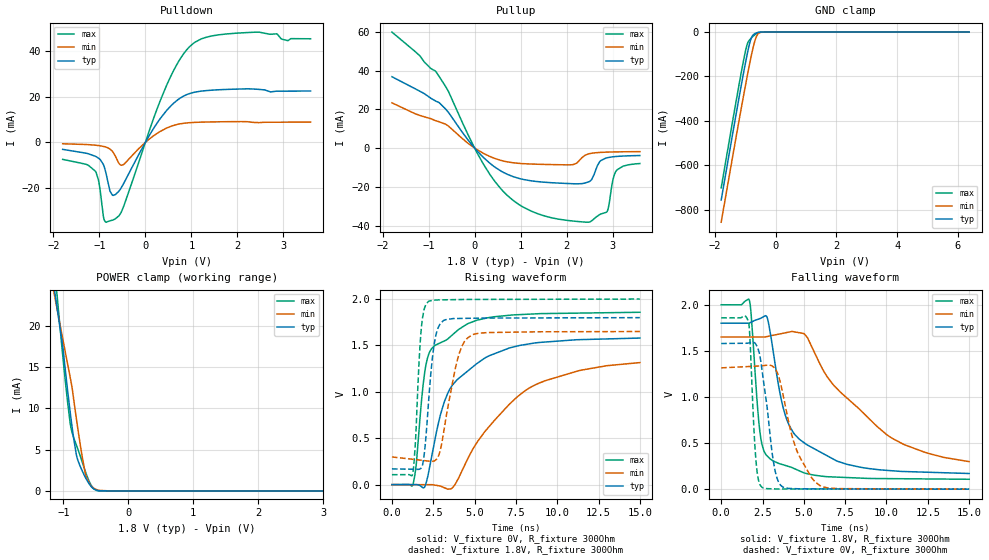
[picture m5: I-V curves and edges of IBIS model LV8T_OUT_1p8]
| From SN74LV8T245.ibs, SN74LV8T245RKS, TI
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[Model]   LV8T_OUT_1p8
Model_type   I/O
Polarity   Non-Inverting
Enable   Active-Low
Vinl = 0.51
Vinh = 1.1
Vmeas = 0.9
Vref = 0
Cref = 2pF
Rref = 100000
|   typ   min   max
C_comp   6.7pF   6.5pF   7pF
[Voltage Range]   1.8   1.65   2
[Temperature Range]   25   125   -40
[Pullup Reference]   1.8   1.65   2
[Pulldown Reference]   0   0   0
[Power Clamp Reference]   1.8   1.65   2
[GND Clamp Reference]   0   0   0
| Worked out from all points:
|   slope of the pulldown table from 0 to 0.27 V, typ, clamps not added: 30.3 ohm
|   slope of the pullup table from 0 to 0.27 V, typ, clamps not added: 41.2 ohm
|   GND clamp passes 1 mA (typ) near -0.56 V on its own axis
|   POWER clamp passes 1 mA (typ) near -0.61 V on its own axis
|   falling waveform, V_fixture 1.8V, R_fixture 300Ohm: 20-80 % time 1.91ns typ, 4.28ns min, 546ps max; typ from 1.8 V to 0.17 V
|   rising waveform, V_fixture 0V, R_fixture 300Ohm: 20-80 % time 2.44ns typ, 3.87ns min, 971ps max; typ from 0 V to 1.58 V
|   rising waveform, V_fixture 1.8V, R_fixture 300Ohm: 20-80 % time 477ps typ, 882ps min, 317ps max; typ from 0.17 V to 1.8 V
|   falling waveform, V_fixture 0V, R_fixture 300Ohm: 20-80 % time 656ps typ, 1.31ns min, 299ps max; typ from 1.58 V to 0 V
[Pulldown]
|   Voltage   I(typ)   I(min)   I(max)
-1.796V   -3.045mA   -600uA     -7.42mA
-1.083V   -6.104mA   -1.23mA    -12.66mA
-1.009V   -7.035mA   -1.406mA   -17.51mA
-893.5mV  -10.69mA   -1.841mA   -33.97mA
-767.5mV  -21.4mA    -2.913mA   -34.28mA
-694mV    -23.17mA   -4.51mA    -33.86mA
-473.5mV  -18.04mA   -9.675mA   -28.07mA
324.5mV   10.45mA    4.819mA    18.3mA
618.5mV   17.21mA    7.455mA    31.63mA
954.5mV   21.33mA    8.616mA    41.74mA
1.962V    23.3mA     9.091mA    47.75mA
3.59V     22.5mA     8.877mA    45.34mA
[GND Clamp]
|   Voltage   I(typ)   I(min)   I(max)
-1.796V   -756.6mA   -856.2mA   -701.6mA
-1.188V   -279.6mA   -382.9mA   -221.3mA
-1.072V   -193.2mA   -296.1mA   -136.2mA
-988mV    -132.9mA   -234.2mA   -80.47mA
-914.5mV  -83.48mA   -181.5mA   -46.74mA
-851.5mV  -47.24mA   -137.9mA   -33.82mA
-799mV    -25.51mA   -103.2mA   -26.25mA
-683.5mV  -6.635mA   -38.29mA   -11.53mA
-631mV    -3.444mA   -18.64mA   -6.502mA
-568mV    -1.185mA   -5.967mA   -2.299mA
-274mV    -10.31nA   -2.458uA   0A
6.372V    0A         0A         0A
[Pullup]
|   Voltage   I(typ)   I(min)   I(max)
-1.796V   36.82mA    23.35mA    59.86mA
-841mV    24.17mA    14.08mA    39.43mA
324.5mV   -7.713mA   -4.277mA   -13.36mA
702.5mV   -13.49mA   -7.102mA   -24.3mA
1.081V    -16.33mA   -8.097mA   -30.81mA
2.131V    -18.42mA   -8.573mA   -37.67mA
2.509V    -17.08mA   -2.833mA   -38.09mA
2.719V    -7.037mA   -2.275mA   -34.36mA
2.886V    -4.992mA   -2.098mA   -32.39mA
3.002V    -4.533mA   -2.025mA   -16.75mA
3.075V    -4.357mA   -1.99mA    -11.82mA
3.59V     -3.877mA   -1.859mA   -7.992mA
[POWER Clamp]
|   Voltage   I(typ)   I(min)   I(max)
-1.796V   61.45mA    51.6mA     74.22mA
-1.188V   27.14mA    25.88mA    30.08mA
-1.103V   22.6mA     22.36mA    24.31mA
-1.093V   22.04mA    21.92mA    23.5mA
-1.009V   17.53mA    18.45mA    16.44mA
-967mV    14.55mA    16.74mA    13.18mA
-883mV    8.87mA     13.32mA    7.694mA
-799mV    4.394mA    8.8mA      5.562mA
-662.5mV  1.684mA    2.226mA    2.411mA
-599.5mV  831uA      918.6uA    1.136mA
-484mV    74.52uA    145.8uA    53.97uA
6.372V    0A         0A         0A
[Ramp]
R_load = 300
|   typ   min   max
dV/dt_r   0.947756/2.43296e-09   0.789158/3.87689e-09   1.11451/9.59874e-10
dV/dt_f   0.977899/1.90392e-09   0.810908/4.28098e-09   1.13551/5.4593e-10
[Falling Waveform]
V_fixture = 1.8V
V_fixture_min = 1.65V
V_fixture_max = 2V
R_fixture = 300Ohm
C_fixture = 0F
|   Time   V(typ)   V(min)   V(max)
0s        1.8V       1.65V      2V
1.701ns   1.801V     1.65V      2.051V
2.357ns   1.851V     1.65V      603mV
2.733ns   1.878V     1.654V     369.1mV
2.975ns   1.689V     1.663V     326.5mV
3.926ns   776.4mV    1.697V     254.8mV
5.125ns   489.2mV    1.664V     171.1mV
6.735ns   330.7mV    1.142V     132.8mV
9.983ns   204.4mV    595.9mV    114.5mV
15ns      169.8mV    298.5mV    107.3mV
[Rising Waveform]
V_fixture = 0V
V_fixture_min = 0V
V_fixture_max = 0V
R_fixture = 300Ohm
C_fixture = 0F
|   Time   V(typ)   V(min)   V(max)
0s        101.7uV    1.708uV    32.48uV
1.269ns   589.5uV    -297.5uV   -85.04uV
1.466ns   665.3uV    -344uV     208.2mV
1.993ns   -20.9mV    -468.3uV   1.222V
2.568ns   452.4mV    -4.419mV   1.495V
2.95ns    762.7mV    -16.71mV   1.53V
3.531ns   1.038V     -46.61mV   1.594V
5.855ns   1.387V     620.6mV    1.8V
8.786ns   1.53V      1.085V     1.841V
15ns      1.58V      1.315V     1.858V
[Rising Waveform]
V_fixture = 1.8V
V_fixture_min = 1.65V
V_fixture_max = 2V
R_fixture = 300Ohm
C_fixture = 0F
|   Time   V(typ)   V(min)   V(max)
0s        169.8mV    298.5mV    107.3mV
1.257ns   165.8mV    273.2mV    116.4mV
1.423ns   165.3mV    269.8mV    460.7mV
1.77ns    180.2mV    262.8mV    1.668V
2.195ns   840.2mV    254.3mV    1.972V
2.487ns   1.422V     252.5mV    1.986V
2.787ns   1.688V     297.9mV    1.991V
4ns       1.791V     1.371V     1.994V
4.809ns   1.793V     1.61V      1.996V
15ns      1.8V       1.65V      2V
[Falling Waveform]
|Gnd
V_fixture = 0V
V_fixture_min = 0V
V_fixture_max = 0V
R_fixture = 300Ohm
C_fixture = 0F
|   Time   V(typ)   V(min)   V(max)
0s        1.58V      1.315V     1.858V
1.66ns    1.585V     1.33V      1.807V
1.729ns   1.588V     1.331V     1.67V
2.102ns   1.57V      1.334V     315.1mV
2.473ns   1.287V     1.339V     19.42mV
3.22ns    236.3mV    1.316V     3.147mV
3.711ns   25.39mV    1.052V     2.139mV
4.551ns   4.927mV    429.9mV    1.983mV
5.984ns   2.804mV    37.73mV    1.715mV
15ns      101.7uV    1.708uV    32.49uV
